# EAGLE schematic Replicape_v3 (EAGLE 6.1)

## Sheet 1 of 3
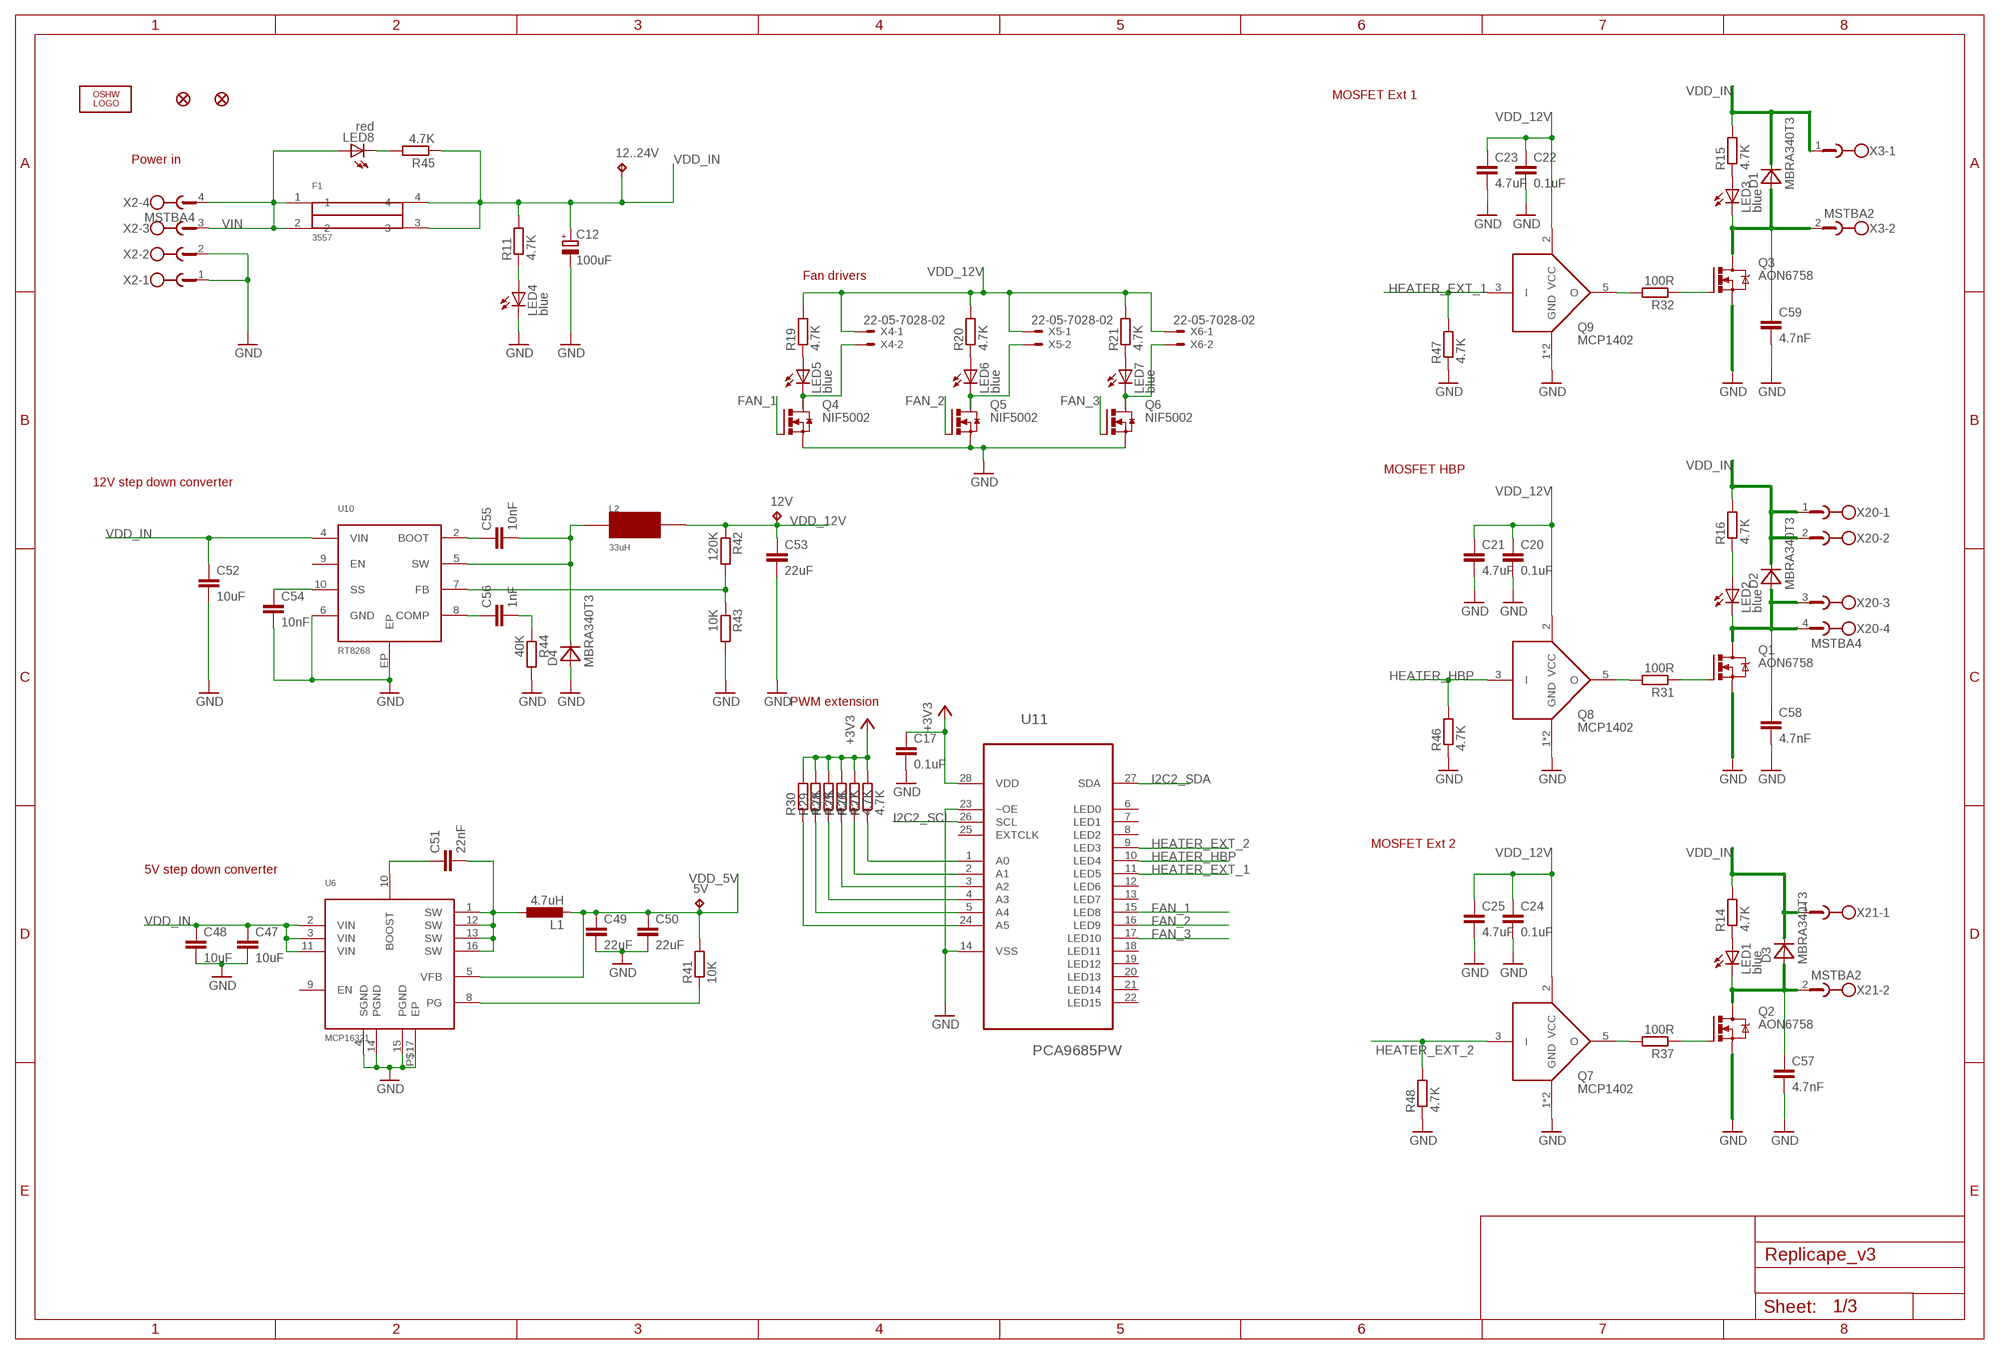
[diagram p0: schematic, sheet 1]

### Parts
5V  TPB1,27  [B1,27]
12..24V  TPB1,27  [B1,27]
12V  TPB1,27  [B1,27]
C12  100uF  CPOL-EU140CLH-0810  [140CLH-0810]
C17  0.1uF  C-EUC0402  [C0402]
C20  0.1uF  C-EUC0402  [C0402]
C21  4.7uF  C-EUC0402  [C0402]
C22  0.1uF  C-EUC0402  [C0402]
C23  4.7uF  C-EUC0402  [C0402]
C24  0.1uF  C-EUC0402  [C0402]
C25  4.7uF  C-EUC0402  [C0402]
C47  10uF  C-EUC1206  [C1206]
C48  10uF  C-EUC1206  [C1206]
C49  22uF  C-EUC0805  [C0805]
C50  22uF  C-EUC0805  [C0805]
C51  22nF  C-EUC0402  [C0402]
C52  10uF  C-EUC1206  [C1206]
C53  22uF  C-EUC0805  [C0805]
C54  10nF  C-EUC0402  [C0402]
C55  10nF  C-EUC0402  [C0402]
C56  1nF  C-EUC0402  [C0402]
C57  4.7nF  C-EUC0402  [C0402]
C58  4.7nF  C-EUC0402  [C0402]
C59  4.7nF  C-EUC0402  [C0402]
D1  MBRA340T3  [SMA]
D2  MBRA340T3  [SMA]
D3  MBRA340T3  [SMA]
D4  MBRA340T3  [SMA]
F1  3557  [3557]
JP1  FIDUCIAL1X2.5  [FIDUCIAL-1X2.5]
JP2  FIDUCIAL1X2.5  [FIDUCIAL-1X2.5]
L1  4.7uH  L-EUVLC  [VLC5020]
L2  33uH  RT8040T330  [NR8040T330]
LED1  blue  LEDCHIP-LED0603  [CHIP-LED0603]
LED2  blue  LEDCHIP-LED0603  [CHIP-LED0603]
LED3  blue  LEDCHIP-LED0603  [CHIP-LED0603]
LED4  blue  LEDCHIP-LED0603  [CHIP-LED0603]
LED5  blue  LEDCHIP-LED0603  [CHIP-LED0603]
LED6  blue  LEDCHIP-LED0603  [CHIP-LED0603]
LED7  blue  LEDCHIP-LED0603  [CHIP-LED0603]
LED8  red  LEDCHIP-LED0603  [CHIP-LED0603]
LOGO1  OSHW_LOGO_FILLX0200-NT  [OSHW_FILLX200_NOTEXT]
Q1  AON6758  [8-DFN-EP-(5X6)]
Q2  AON6758  [8-DFN-EP-(5X6)]
Q3  AON6758  [8-DFN-EP-(5X6)]
Q4  NIF5002  N-HEXFET-2D_SOT232-  [SOT223]
Q5  NIF5002  N-HEXFET-2D_SOT232-  [SOT223]
Q6  NIF5002  N-HEXFET-2D_SOT232-  [SOT223]
Q7  MCP1402  [SOT23-5L]
Q8  MCP1402  [SOT23-5L]
Q9  MCP1402  [SOT23-5L]
R11  4.7K  R-EU_R0402  [R0402]
R14  4.7K  R-EU_R0402  [R0402]
R15  4.7K  R-EU_R0402  [R0402]
R16  4.7K  R-EU_R0402  [R0402]
R19  4.7K  R-EU_R0402  [R0402]
R20  4.7K  R-EU_R0402  [R0402]
R21  4.7K  R-EU_R0402  [R0402]
R25  4.7K  R-EU_R0402  [R0402]
R26  4.7K  R-EU_R0402  [R0402]
R27  4.7K  R-EU_R0402  [R0402]
R28  4.7K  R-EU_R0402  [R0402]
R29  4.7K  R-EU_R0402  [R0402]
R30  4.7K  R-EU_R0402  [R0402]
R31  100R  R-EU_R0402  [R0402]
R32  100R  R-EU_R0402  [R0402]
R37  100R  R-EU_R0402  [R0402]
R41  10K  R-EU_R0402  [R0402]
R42  120K  R-EU_R0402  [R0402]
R43  10K  R-EU_R0402  [R0402]
R44  40K  R-EU_R0402  [R0402]
R45  4.7K  R-EU_R0402  [R0402]
R46  4.7K  R-EU_R0402  [R0402]
R47  4.7K  R-EU_R0402  [R0402]
R48  4.7K  R-EU_R0402  [R0402]
U6  MCP16321  [QFN-16]
U10  RT8268  [MSOP10]
U11  PCA9685PW  [SOP65P640X110-28N]
X2  MSTBA4  [MSTBA4]
X3  MSTBA2  [MSTBA2]
X4  22-05-7028-02  [7395-02]
X5  22-05-7028-02  [7395-02]
X6  22-05-7028-02  [7395-02]
X20  MSTBA4  [MSTBA4]
X21  MSTBA2  [MSTBA2]

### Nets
+3V3: C17.1 R25.2 R26.2 R27.2 R28.2 R29.2 R30.2 U11.28(VDD) ; also sheet 2,3
FAN_1: Q4.1(G) U11.15(LED8)
FAN_2: Q5.1(G) U11.16(LED9)
FAN_3: Q6.1(G) U11.17(LED10)
GND: C12.- C17.2 C20.2 C21.2 C22.2 C23.2 C24.2 C25.2 C47.2 C48.2 C49.2 C50.2 C52.2 C53.2 C54.2 C57.2 C58.2 C59.2 D4.A LED4.C Q1.1(S) Q1.2(S) Q1.3(S) Q2.1(S) Q2.2(S) Q2.3(S) Q3.1(S) Q3.2(S) Q3.3(S) Q4.3(S) Q5.3(S) Q6.3(S) Q7.1(GND) Q7.4(GND) Q8.1(GND) Q8.4(GND) Q9.1(GND) Q9.4(GND) R43.2 R44.2 R46.1 R47.1 R48.1 U6.4(SGND) U6.14(PGND) U6.15(PGND) U6.P$17(EP) U10.6(GND) U10.EP U11.14(VSS) U11.23(~OE) X2.1 X2.2 ; also sheet 2,3
HEATER_EXT_1: Q9.3(I) R47.2 U11.11(LED5)
HEATER_EXT_2: Q7.3(I) R48.2 U11.9(LED3)
HEATER_HBP: Q8.3(I) R46.2 U11.10(LED4)
I2C2_SCL: U11.26(SCL) ; also sheet 2
I2C2_SDA: U11.27(SDA) ; also sheet 2
N$8: LED8.C R45.2
N$9: LED5.A R19.1
N$21: Q9.5(O) R32.2
N$23: Q2.4(G) R37.1
N$41: Q7.5(O) R37.2
N$58: R27.1 U11.1(A0)
N$59: R26.1 U11.2(A1)
N$60: Q1.4(G) R31.1
N$61: Q8.5(O) R31.2
N$64: C57.1 D3.A LED1.C Q2.5(D) Q2.6(D) Q2.7(D) Q2.8(D) Q2.TH(D) X21.2
N$76: R25.1 U11.3(A2)
N$94: R28.1 U11.4(A3)
N$95: R29.1 U11.5(A4)
N$96: LED4.A R11.1
N$112: R30.1 U11.24(A5)
N$114: LED7.C Q6.2(D) Q6.4(D) X6.2
N$115: LED6.C Q5.2(D) Q5.4(D) X5.2
N$116: LED5.C Q4.2(D) Q4.4(D) X4.2
N$117: LED6.A R20.1
N$118: LED7.A R21.1
N$127: LED3.A R15.1
N$128: C51.1 U6.10(BOOST)
N$129: LED1.A R14.1
N$130: LED2.A R16.1
N$133: Q3.4(G) R32.1
N$233: R42.2 R43.1 U10.7(FB)
N$234: C59.1 D1.A LED3.C Q3.5(D) Q3.6(D) Q3.7(D) Q3.8(D) Q3.TH(D) X3.2
N$238: C55.2 D4.C L2.P$2 U10.5(SW)
N$239: R41.1 U6.8(PG)
N$242: C58.1 D2.A LED2.C Q1.5(D) Q1.6(D) Q1.7(D) Q1.8(D) Q1.TH(D) X20.3 X20.4
N$243: C54.1 U10.10(SS)
N$244: C56.1 U10.8(COMP)
N$245: C55.1 U10.2(BOOT)
N$246: C56.2 R44.1
SW: C51.2 L1.1 U6.1(SW) U6.12(SW) U6.13(SW) U6.16(SW)
VDD_5V: 5V.TP C49.1 C50.1 L1.2 R41.2 U6.5(VFB) ; also sheet 2
VDD_12V: 12V.TP C20.1 C21.1 C22.1 C23.1 C24.1 C25.1 C53.1 L2.P$1 Q7.2(VCC) Q8.2(VCC) Q9.2(VCC) R19.2 R20.2 R21.2 R42.1 X4.1 X5.1 X6.1
VDD_IN: 12..24V.TP C12.+ C47.1 C48.1 C52.1 D1.C D2.C D3.C F1.3 F1.4 R11.2 R14.2 R15.2 R16.2 R45.1 U6.2(VIN) U6.3(VIN) U6.11(VIN) U10.4(VIN) X3.1 X20.1 X20.2 X21.1 ; also sheet 3
VIN: F1.1 F1.2 LED8.A X2.3 X2.4
Unconnected: U6.9(EN) U10.9(EN) U11.6(LED0) U11.7(LED1) U11.8(LED2) U11.12(LED6) U11.13(LED7) U11.18(LED11) U11.19(LED12) U11.20(LED13) U11.21(LED14) U11.22(LED15) U11.25(EXTCLK)

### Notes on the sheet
- MOSFET Ext 1
- Power in
- Fan drivers
- MOSFET HBP
- 12V step down converter
- PWM extension
- MOSFET Ext 2
- 5V step down converter

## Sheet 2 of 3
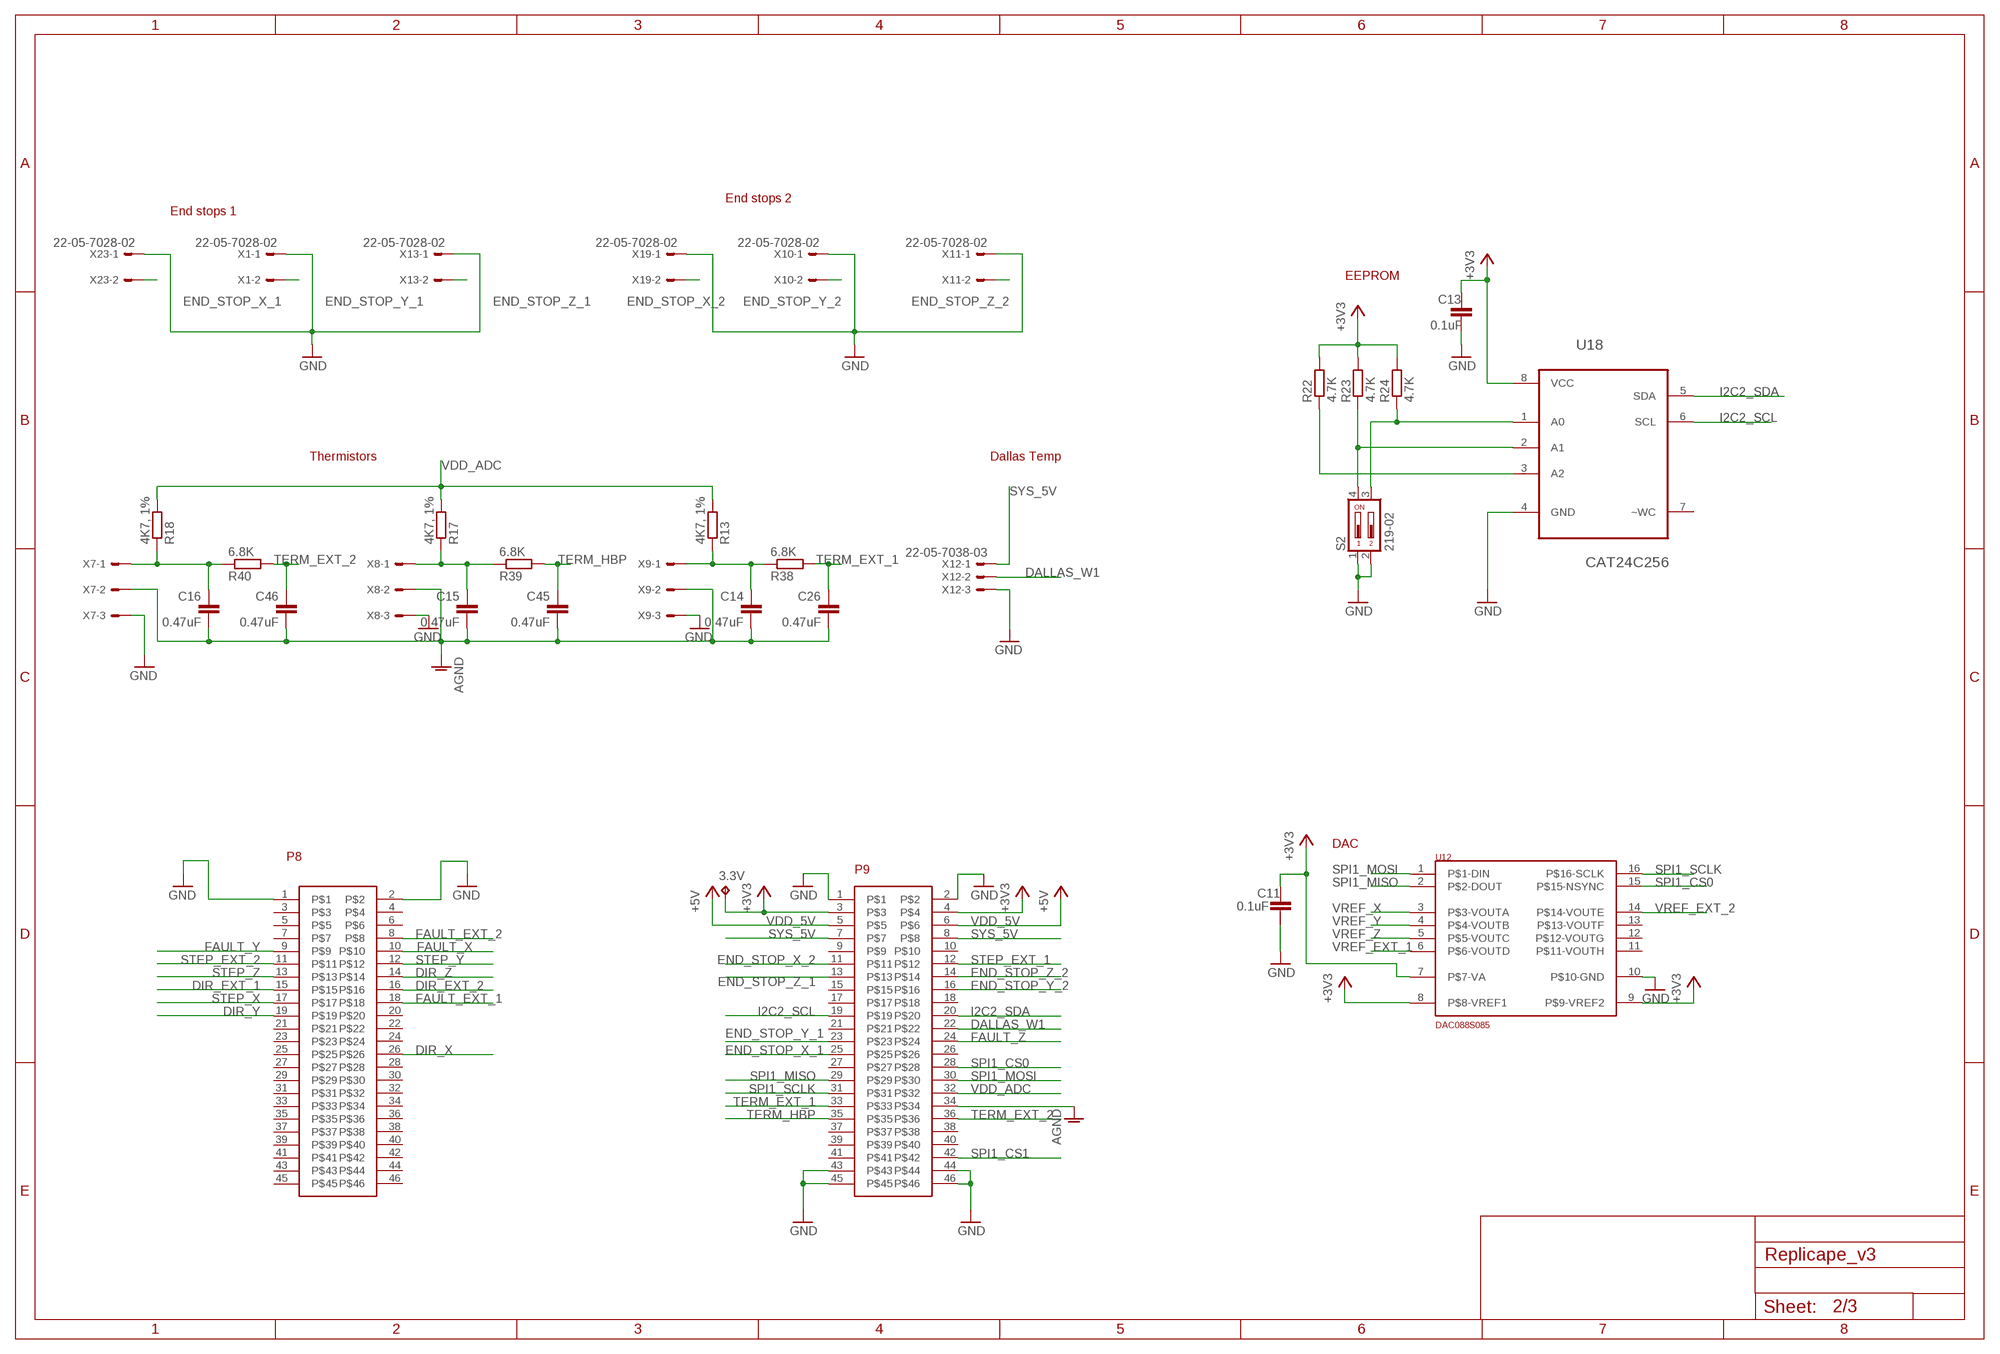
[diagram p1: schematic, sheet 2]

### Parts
3.3V  TPB1,27  [B1,27]
C11  0.1uF  C-EUC0402  [C0402]
C13  0.1uF  C-EUC0402  [C0402]
C14  0.47uF  C-EUC0402  [C0402]
C15  0.47uF  C-EUC0402  [C0402]
C16  0.47uF  C-EUC0402  [C0402]
C26  0.47uF  C-EUC0402  [C0402]
C45  0.47uF  C-EUC0402  [C0402]
C46  0.47uF  C-EUC0402  [C0402]
P9-EXPANSION_A  BEAGLE_EXT9  [2X23]
P9-EXPANSION_A1  BEAGLE_EXT9  [2X23]
R13  4K7, 1%  R-EU_R0402  [R0402]
R17  4K7, 1%  R-EU_R0402  [R0402]
R18  4K7, 1%  R-EU_R0402  [R0402]
R22  4.7K  R-EU_R0402  [R0402]
R23  4.7K  R-EU_R0402  [R0402]
R24  4.7K  R-EU_R0402  [R0402]
R38  6.8K  R-EU_R0402  [R0402]
R39  6.8K  R-EU_R0402  [R0402]
R40  6.8K  R-EU_R0402  [R0402]
S2  219-02  [CTS-219-02]
U12  DAC088S085  [TSSOP-16]
U18  CAT24C256  [SOIC127P600X175-8N]
X1  22-05-7028-02  [7395-02]
X7  22-05-7038-03  [7395-03]
X8  22-05-7038-03  [7395-03]
X9  22-05-7038-03  [7395-03]
X10  22-05-7028-02  [7395-02]
X11  22-05-7028-02  [7395-02]
X12  22-05-7038-03  [7395-03]
X13  22-05-7028-02  [7395-02]
X19  22-05-7028-02  [7395-02]
X23  22-05-7028-02  [7395-02]

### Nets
+3V3: 3.3V.TP C11.1 C13.1 P9-EXPANSION_A.3 P9-EXPANSION_A.4 R22.2 R23.2 R24.2 U12.7(P$7-VA) U12.8(P$8-VREF1) U12.9(P$9-VREF2) U18.8(VCC) ; also sheet 1,3
AGND: C14.2 C15.2 C16.2 C26.2 C45.2 C46.2 P9-EXPANSION_A.34 X7.2 X8.2 X9.2
DALLAS_W1: P9-EXPANSION_A.22 X12.2
DIR_EXT_1: P9-EXPANSION_A1.15 ; also sheet 3
DIR_EXT_2: P9-EXPANSION_A1.16 ; also sheet 3
DIR_X: P9-EXPANSION_A1.26 ; also sheet 3
DIR_Y: P9-EXPANSION_A1.19 ; also sheet 3
DIR_Z: P9-EXPANSION_A1.14 ; also sheet 3
END_STOP_X_1: P9-EXPANSION_A.25 X23.2
END_STOP_X_2: P9-EXPANSION_A.11 X19.2
END_STOP_Y_1: P9-EXPANSION_A.23 X1.2
END_STOP_Y_2: P9-EXPANSION_A.16 X10.2
END_STOP_Z_1: P9-EXPANSION_A.13 X13.2
END_STOP_Z_2: P9-EXPANSION_A.14 X11.2
FAULT_EXT_1: P9-EXPANSION_A1.18 ; also sheet 3
FAULT_EXT_2: P9-EXPANSION_A1.8 ; also sheet 3
FAULT_X: P9-EXPANSION_A1.10 ; also sheet 3
FAULT_Y: P9-EXPANSION_A1.9 ; also sheet 3
FAULT_Z: P9-EXPANSION_A.24 ; also sheet 3
GND: C11.2 C13.2 P9-EXPANSION_A1.1 P9-EXPANSION_A1.2 P9-EXPANSION_A.1 P9-EXPANSION_A.2 P9-EXPANSION_A.43 P9-EXPANSION_A.44 P9-EXPANSION_A.45 P9-EXPANSION_A.46 S2.1 S2.2 U12.10(P$10-GND) U18.4(GND) X1.1 X7.3 X8.3 X9.3 X10.1 X11.1 X12.3 X13.1 X19.1 X23.1 ; also sheet 1,3
I2C2_SCL: P9-EXPANSION_A.19 U18.6(SCL) ; also sheet 1
I2C2_SDA: P9-EXPANSION_A.20 U18.5(SDA) ; also sheet 1
N$147: R24.1 S2.3 U18.1(A0)
N$148: R23.1 S2.4 U18.2(A1)
N$149: R22.1 U18.3(A2)
N$237: C14.1 R13.1 R38.1 X9.1
N$240: C16.1 R18.1 R40.1 X7.1
N$241: C15.1 R17.1 R39.1 X8.1
SPI1_CS0: P9-EXPANSION_A.28 U12.15(P$15-NSYNC)
SPI1_CS1: P9-EXPANSION_A.42 ; also sheet 3
SPI1_MISO: P9-EXPANSION_A.29 U12.2(P$2-DOUT)
SPI1_MOSI: P9-EXPANSION_A.30 U12.1(P$1-DIN) ; also sheet 3
SPI1_SCLK: P9-EXPANSION_A.31 U12.16(P$16-SCLK) ; also sheet 3
STEP_EXT_1: P9-EXPANSION_A.12 ; also sheet 3
STEP_EXT_2: P9-EXPANSION_A1.11 ; also sheet 3
STEP_X: P9-EXPANSION_A1.17 ; also sheet 3
STEP_Y: P9-EXPANSION_A1.12 ; also sheet 3
STEP_Z: P9-EXPANSION_A1.13 ; also sheet 3
SYS_5V: P9-EXPANSION_A.7 P9-EXPANSION_A.8 X12.1
TERM_EXT_1: C26.1 P9-EXPANSION_A.33 R38.2
TERM_EXT_2: C46.1 P9-EXPANSION_A.36 R40.2
TERM_HBP: C45.1 P9-EXPANSION_A.35 R39.2
VDD_5V: P9-EXPANSION_A.5 P9-EXPANSION_A.6 ; supply symbol labelled +5V ; also sheet 1
VDD_ADC: P9-EXPANSION_A.32 R13.2 R17.2 R18.2
VREF_EXT_1: U12.6(P$6-VOUTD) ; also sheet 3
VREF_EXT_2: U12.14(P$14-VOUTE) ; also sheet 3
VREF_X: U12.3(P$3-VOUTA) ; also sheet 3
VREF_Y: U12.4(P$4-VOUTB) ; also sheet 3
VREF_Z: U12.5(P$5-VOUTC) ; also sheet 3
Unconnected: P9-EXPANSION_A1.3 P9-EXPANSION_A1.4 P9-EXPANSION_A1.5 P9-EXPANSION_A1.6 P9-EXPANSION_A1.7 P9-EXPANSION_A1.20 P9-EXPANSION_A1.21 P9-EXPANSION_A1.22 P9-EXPANSION_A1.23 P9-EXPANSION_A1.24 P9-EXPANSION_A1.25 P9-EXPANSION_A1.27 P9-EXPANSION_A1.28 P9-EXPANSION_A1.29 P9-EXPANSION_A1.30 P9-EXPANSION_A1.31 P9-EXPANSION_A1.32 P9-EXPANSION_A1.33 P9-EXPANSION_A1.34 P9-EXPANSION_A1.35 P9-EXPANSION_A1.36 P9-EXPANSION_A1.37 P9-EXPANSION_A1.38 P9-EXPANSION_A1.39 P9-EXPANSION_A1.40 P9-EXPANSION_A1.41 P9-EXPANSION_A1.42 P9-EXPANSION_A1.43 P9-EXPANSION_A1.44 P9-EXPANSION_A1.45 P9-EXPANSION_A1.46 P9-EXPANSION_A.9 P9-EXPANSION_A.10 P9-EXPANSION_A.15 P9-EXPANSION_A.17 P9-EXPANSION_A.18 P9-EXPANSION_A.21 P9-EXPANSION_A.26 P9-EXPANSION_A.27 P9-EXPANSION_A.37 P9-EXPANSION_A.38 P9-EXPANSION_A.39 P9-EXPANSION_A.40 P9-EXPANSION_A.41 U12.11(P$11-VOUTH) U12.12(P$12-VOUTG) U12.13(P$13-VOUTF) U18.7(~WC)

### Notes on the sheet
- End stops 2
- End stops 1
- EEPROM
- Thermistors | Dallas Temp
- DAC
- P8
- P9

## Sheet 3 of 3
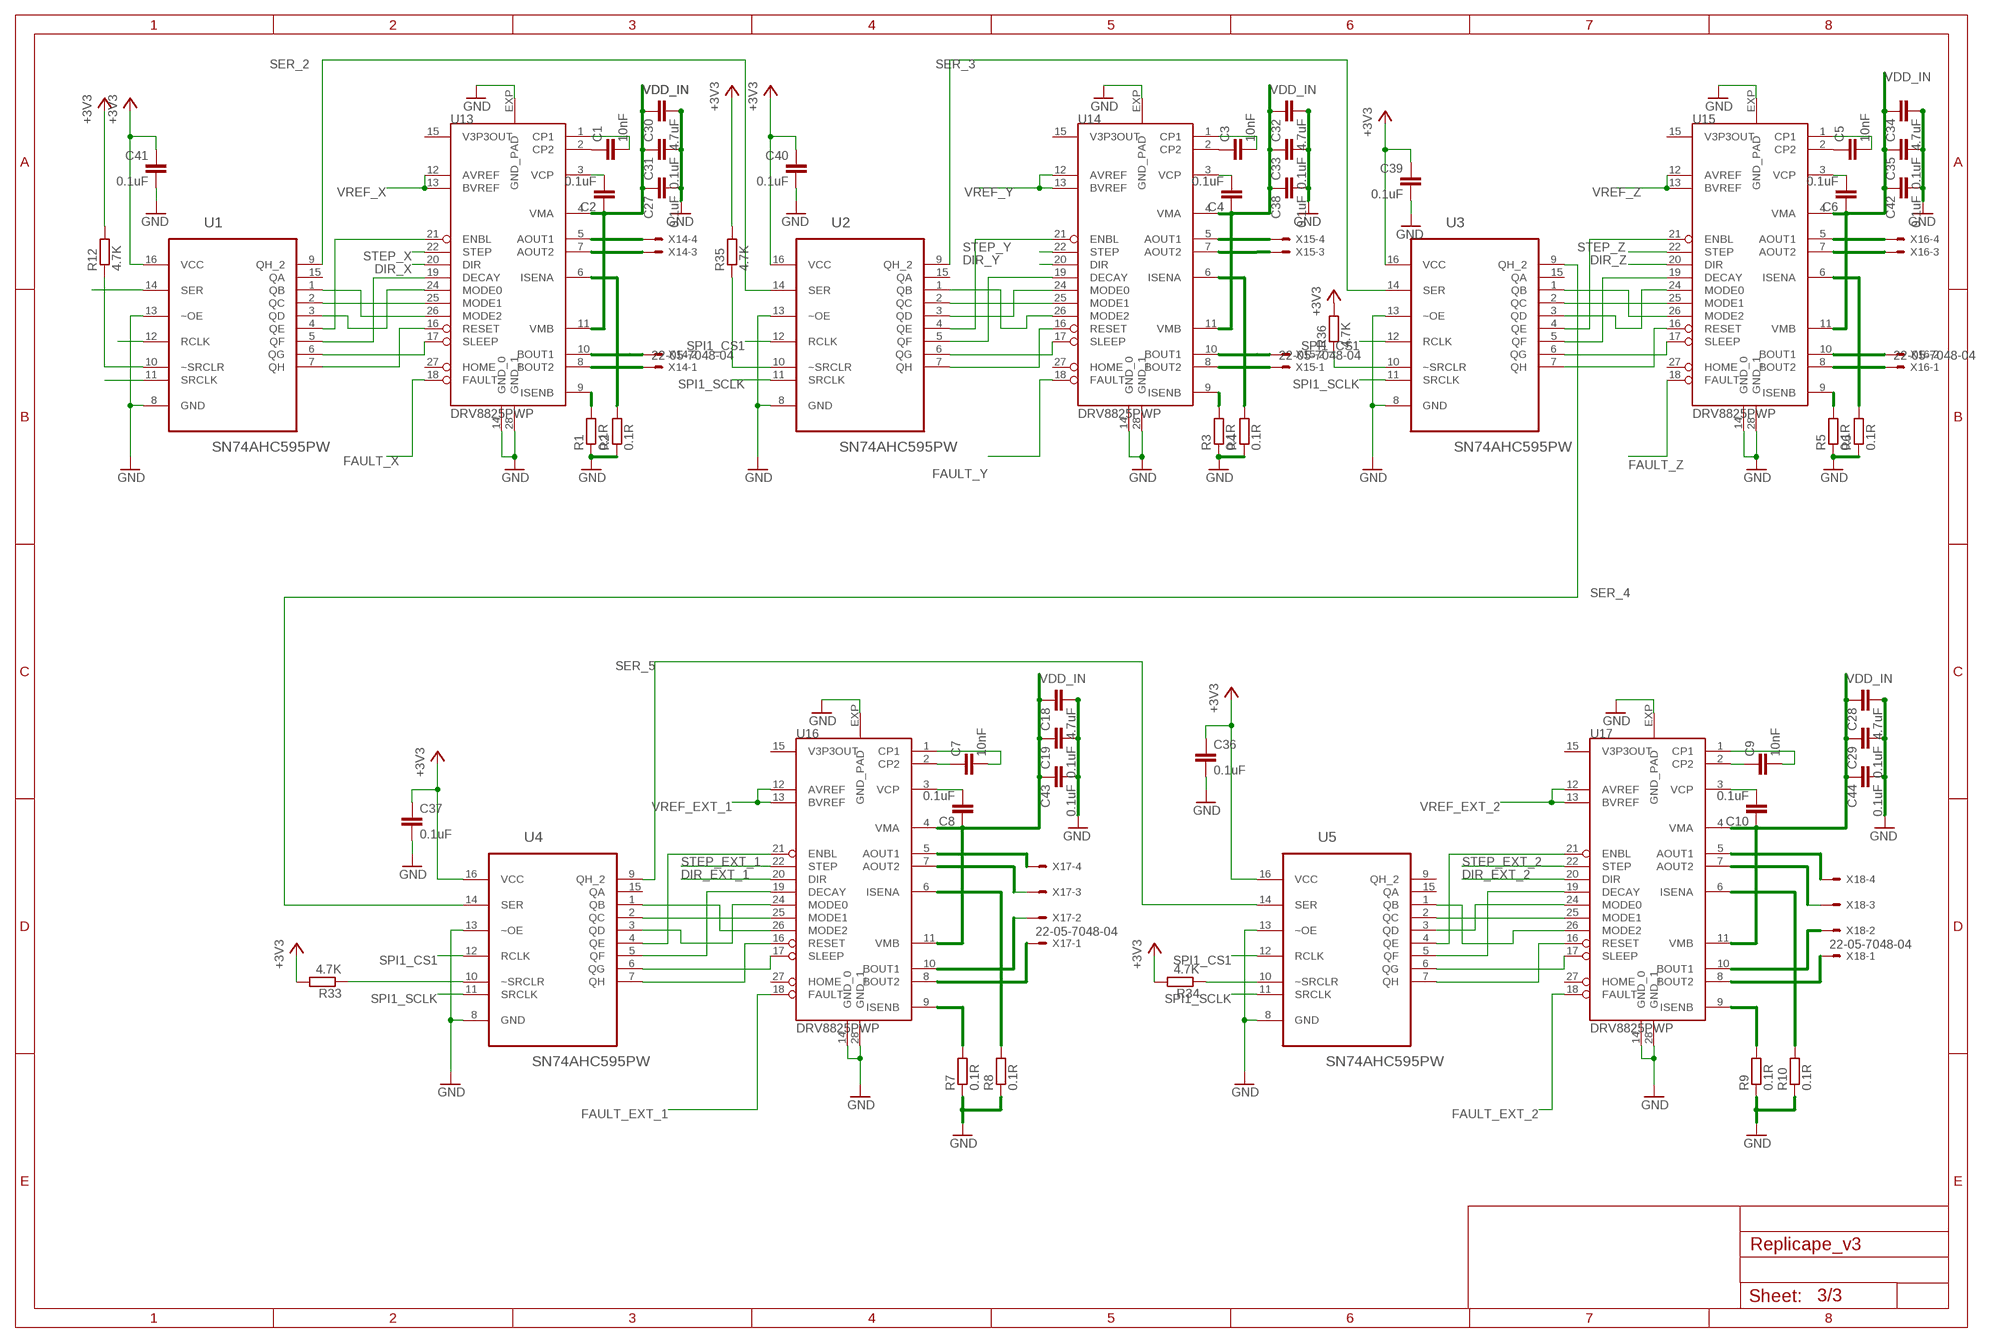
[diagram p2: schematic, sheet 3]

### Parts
C1  10nF  C-EUC0402  [C0402]
C2  0.1uF  C-EUC0402  [C0402]
C3  10nF  C-EUC0402  [C0402]
C4  0.1uF  C-EUC0402  [C0402]
C5  10nF  C-EUC0402  [C0402]
C6  0.1uF  C-EUC0402  [C0402]
C7  10nF  C-EUC0402  [C0402]
C8  0.1uF  C-EUC0402  [C0402]
C9  10nF  C-EUC0402  [C0402]
C10  0.1uF  C-EUC0402  [C0402]
C18  4.7uF  C-EUC0603  [C0603]
C19  0.1uF  C-EUC0402  [C0402]
C27  0.1uF  C-EUC0402  [C0402]
C28  4.7uF  C-EUC0603  [C0603]
C29  0.1uF  C-EUC0402  [C0402]
C30  4.7uF  C-EUC0603  [C0603]
C31  0.1uF  C-EUC0402  [C0402]
C32  4.7uF  C-EUC0603  [C0603]
C33  0.1uF  C-EUC0402  [C0402]
C34  4.7uF  C-EUC0603  [C0603]
C35  0.1uF  C-EUC0402  [C0402]
C36  0.1uF  C-EUC0402  [C0402]
C37  0.1uF  C-EUC0402  [C0402]
C38  0.1uF  C-EUC0402  [C0402]
C39  0.1uF  C-EUC0402  [C0402]
C40  0.1uF  C-EUC0402  [C0402]
C41  0.1uF  C-EUC0402  [C0402]
C42  0.1uF  C-EUC0402  [C0402]
C43  0.1uF  C-EUC0402  [C0402]
C44  0.1uF  C-EUC0402  [C0402]
R1  0.1R  R-EU_R0805  [R0805]
R2  0.1R  R-EU_R0805  [R0805]
R3  0.1R  R-EU_R0805  [R0805]
R4  0.1R  R-EU_R0805  [R0805]
R5  0.1R  R-EU_R0805  [R0805]
R6  0.1R  R-EU_R0805  [R0805]
R7  0.1R  R-EU_R0805  [R0805]
R8  0.1R  R-EU_R0805  [R0805]
R9  0.1R  R-EU_R0805  [R0805]
R10  0.1R  R-EU_R0805  [R0805]
R12  4.7K  R-EU_R0402  [R0402]
R33  4.7K  R-EU_R0402  [R0402]
R34  4.7K  R-EU_R0402  [R0402]
R35  4.7K  R-EU_R0402  [R0402]
R36  4.7K  R-EU_R0402  [R0402]
U1  SN74AHC595PW  [SOP65P640X120-16N]
U2  SN74AHC595PW  [SOP65P640X120-16N]
U3  SN74AHC595PW  [SOP65P640X120-16N]
U4  SN74AHC595PW  [SOP65P640X120-16N]
U5  SN74AHC595PW  [SOP65P640X120-16N]
U13  DRV8825PWP  [TSSOP-28]
U14  DRV8825PWP  [TSSOP-28]
U15  DRV8825PWP  [TSSOP-28]
U16  DRV8825PWP  [TSSOP-28]
U17  DRV8825PWP  [TSSOP-28]
X14  22-05-7048-04  [7395-04]
X15  22-05-7048-04  [7395-04]
X16  22-05-7048-04  [7395-04]
X17  22-05-7048-04  [7395-04]
X18  22-05-7048-04  [7395-04]

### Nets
+3V3: C36.1 C37.1 C39.1 C40.1 C41.1 R12.2 R33.2 R34.2 R35.2 R36.2 U1.16(VCC) U2.16(VCC) U3.16(VCC) U4.16(VCC) U5.16(VCC) ; also sheet 1,2
DIR_EXT_1: U16.20(DIR) ; also sheet 2
DIR_EXT_2: U17.20(DIR) ; also sheet 2
DIR_X: U13.20(DIR) ; also sheet 2
DIR_Y: U14.20(DIR) ; also sheet 2
DIR_Z: U15.20(DIR) ; also sheet 2
EXT1_NENABLE: U4.4(QE) U16.21(ENBL)
EXT1_NSLEEP: U4.6(QG) U16.17(SLEEP)
FAULT_EXT_1: U16.18(FAULT) ; also sheet 2
FAULT_EXT_2: U17.18(FAULT) ; also sheet 2
FAULT_X: U13.18(FAULT) ; also sheet 2
FAULT_Y: U14.18(FAULT) ; also sheet 2
FAULT_Z: U15.18(FAULT) ; also sheet 2
GND: C18.2 C19.2 C27.2 C28.2 C29.2 C30.2 C31.2 C32.2 C33.2 C34.2 C35.2 C36.2 C37.2 C38.2 C39.2 C40.2 C41.2 C42.2 C43.2 C44.2 R1.1 R2.1 R3.1 R4.1 R5.1 R6.1 R7.1 R8.1 R9.1 R10.1 U1.8(GND) U1.13(~OE) U2.8(GND) U2.13(~OE) U3.8(GND) U3.13(~OE) U4.8(GND) U4.13(~OE) U5.8(GND) U5.13(~OE) U13.14(GND_0) U13.28(GND_1) U13.EXP(GND_PAD) U14.14(GND_0) U14.28(GND_1) U14.EXP(GND_PAD) U15.14(GND_0) U15.28(GND_1) U15.EXP(GND_PAD) U16.14(GND_0) U16.28(GND_1) U16.EXP(GND_PAD) U17.14(GND_0) U17.28(GND_1) U17.EXP(GND_PAD) ; also sheet 1,2
N$1: U5.1(QB) U17.26(MODE2)
N$2: U5.3(QD) U17.24(MODE0)
N$3: U5.7(QH) U17.16(RESET)
N$4: U4.7(QH) U16.16(RESET)
N$5: U4.3(QD) U16.24(MODE0)
N$6: U4.1(QB) U16.26(MODE2)
N$7: U3.7(QH) U15.16(RESET)
N$11: U3.3(QD) U15.24(MODE0)
N$12: U3.1(QB) U15.26(MODE2)
N$13: U2.7(QH) U14.16(RESET)
N$14: U2.1(QB) U14.26(MODE2)
N$15: U2.3(QD) U14.24(MODE0)
N$16: C1.1 U13.2(CP2)
N$17: C1.2 U13.1(CP1)
N$18: R1.2 U13.9(ISENB)
N$19: R2.2 U13.6(ISENA)
N$20: U1.7(QH) U13.16(RESET)
N$22: C2.2 U13.3(VCP)
N$24: U1.1(QB) U13.26(MODE2)
N$25: U1.3(QD) U13.24(MODE0)
N$26: U2.5(QF) U14.19(DECAY)
N$27: U3.5(QF) U15.19(DECAY)
N$28: U5.5(QF) U17.19(DECAY)
N$29: U4.5(QF) U16.19(DECAY)
N$34: C3.1 U14.2(CP2)
N$35: C3.2 U14.1(CP1)
N$36: R3.2 U14.9(ISENB)
N$37: R4.2 U14.6(ISENA)
N$38: C4.2 U14.3(VCP)
N$52: C5.1 U15.2(CP2)
N$53: C5.2 U15.1(CP1)
N$54: R5.2 U15.9(ISENB)
N$55: R6.2 U15.6(ISENA)
N$56: C6.2 U15.3(VCP)
N$62: U4.2(QC) U16.25(MODE1)
N$70: C7.1 U16.2(CP2)
N$71: C7.2 U16.1(CP1)
N$72: R7.2 U16.9(ISENB)
N$73: R8.2 U16.6(ISENA)
N$74: C8.2 U16.3(VCP)
N$80: U5.2(QC) U17.25(MODE1)
N$83: U5.6(QG) U17.17(SLEEP)
N$88: C9.1 U17.2(CP2)
N$89: C9.2 U17.1(CP1)
N$90: R9.2 U17.9(ISENB)
N$91: R10.2 U17.6(ISENA)
N$92: C10.2 U17.3(VCP)
N$93: U5.4(QE) U17.21(ENBL)
N$97: R12.1 U1.10(~SRCLR)
N$98: R33.1 U4.10(~SRCLR)
N$99: R34.1 U5.10(~SRCLR)
N$100: R35.1 U2.10(~SRCLR)
N$101: R36.1 U3.10(~SRCLR)
SER_2: U1.9(QH_2) U2.14(SER)
SER_3: U2.9(QH_2) U3.14(SER)
SER_4: U3.9(QH_2) U4.14(SER)
SER_5: U4.9(QH_2) U5.14(SER)
SPI1_CS1: U1.12(RCLK) U2.12(RCLK) U3.12(RCLK) U4.12(RCLK) U5.12(RCLK) ; also sheet 2
SPI1_MOSI: U1.14(SER) ; also sheet 2
SPI1_SCLK: U1.11(SRCLK) U2.11(SRCLK) U3.11(SRCLK) U4.11(SRCLK) U5.11(SRCLK) ; also sheet 2
STEP1_EXT1: U16.5(AOUT1) X17.4
STEP1_EXT2: U17.5(AOUT1) X18.4
STEP1_X: U13.5(AOUT1) X14.4
STEP1_Y: U14.5(AOUT1) X15.4
STEP1_Z: U15.5(AOUT1) X16.4
STEP2_EXT1: U16.7(AOUT2) X17.3
STEP2_EXT2: U17.7(AOUT2) X18.3
STEP2_X: U13.7(AOUT2) X14.3
STEP2_Y: U14.7(AOUT2) X15.3
STEP2_Z: U15.7(AOUT2) X16.3
STEP3_EXT1: U16.10(BOUT1) X17.2
STEP3_EXT2: U17.10(BOUT1) X18.2
STEP3_X: U13.10(BOUT1) X14.2
STEP3_Y: U14.10(BOUT1) X15.2
STEP3_Z: U15.10(BOUT1) X16.2
STEP4_EXT1: U16.8(BOUT2) X17.1
STEP4_EXT2: U17.8(BOUT2) X18.1
STEP4_X: U13.8(BOUT2) X14.1
STEP4_Y: U14.8(BOUT2) X15.1
STEP4_Z: U15.8(BOUT2) X16.1
STEP_EXT_1: U16.22(STEP) ; also sheet 2
STEP_EXT_2: U17.22(STEP) ; also sheet 2
STEP_X: U13.22(STEP) ; also sheet 2
STEP_Y: U14.22(STEP) ; also sheet 2
STEP_Z: U15.22(STEP) ; also sheet 2
VDD_IN: C2.1 C4.1 C6.1 C8.1 C10.1 C18.1 C19.1 C27.1 C28.1 C29.1 C30.1 C31.1 C32.1 C33.1 C34.1 C35.1 C38.1 C42.1 C43.1 C44.1 U13.4(VMA) U13.11(VMB) U14.4(VMA) U14.11(VMB) U15.4(VMA) U15.11(VMB) U16.4(VMA) U16.11(VMB) U17.4(VMA) U17.11(VMB) ; also sheet 1
VREF_EXT_1: U16.12(AVREF) U16.13(BVREF) ; also sheet 2
VREF_EXT_2: U17.12(AVREF) U17.13(BVREF) ; also sheet 2
VREF_X: U13.12(AVREF) U13.13(BVREF) ; also sheet 2
VREF_Y: U14.12(AVREF) U14.13(BVREF) ; also sheet 2
VREF_Z: U15.12(AVREF) U15.13(BVREF) ; also sheet 2
X_DECAY: U1.5(QF) U13.19(DECAY)
X_ENABLE: U1.4(QE) U13.21(ENBL)
X_MODE1: U1.2(QC) U13.25(MODE1)
X_SLEEP: U1.6(QG) U13.17(SLEEP)
Y_ENABLE: U2.4(QE) U14.21(ENBL)
Y_MODE1: U2.2(QC) U14.25(MODE1)
Y_SLEEP: U2.6(QG) U14.17(SLEEP)
Z_ENABLE: U3.4(QE) U15.21(ENBL)
Z_MODE1: U3.2(QC) U15.25(MODE1)
Z_SLEEP: U3.6(QG) U15.17(SLEEP)
Unconnected: U1.15(QA) U2.15(QA) U3.15(QA) U4.15(QA) U5.9(QH_2) U5.15(QA) U13.15(V3P3OUT) U13.27(HOME) U14.15(V3P3OUT) U14.27(HOME) U15.15(V3P3OUT) U15.27(HOME) U16.15(V3P3OUT) U16.27(HOME) U17.15(V3P3OUT) U17.27(HOME)

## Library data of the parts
3.3V 5V 12..24V 12V = testpad:TP: Test pad
C1-C11 C13-C59 = rcl:C-EU: CAPACITOR, European symbol
C12 = rcl:CPOL-EU: POLARIZED CAPACITOR, European symbol
D1-D4 = diode:MBRA340T3: Surface Mount Schottky Power Rectifier
F1 = SparkFun:3557
JP1 JP2 = SparkFun:FIDUCIAL: Fiducial Alignment Points
L1 = resistor:L-EU: INDUCTOR, European symbol
L2 = SparkFun:RT8040T330
LED1-LED8 = led:LED: LED
LOGO1 = ohw-logo:OSHW_LOGO_FILL
P9-EXPANSION_A P9-EXPANSION_A1 = custom:BEAGLE_EXT9
Q1-Q3 = transistor-power:AON6758
Q4-Q6 = transistor-power:N-HEXFET-2D_?-*: HEXFET® Power MOSFET 2 Drain connects http://www.irf.com/product-info/datasheets/data/irll014n.pdf
Q7-Q9 = microchip-6:MCP1402: MOSFET driver
R1-R48 = rcl:R-EU_: RESISTOR, European symbol
S2 = switch-dil:219-02*: Surface Mount DIP Switch Series 219 SMT CTS Electronic Components Sourc: www.ctscorp.com; OC_FARNELL: unknown; OC_NEWARK: unknown
U1-U5 = sn74hc595:SN74AHC595PW: 8 bit shift registers with 3-state output registers; MPN: SN74AHC595PW; OC_FARNELL: 1741463; OC_NEWARK: 50R5930; PACKAGE: TSSOP-16; SUPPLIER: Texas Instruments
U6 = SparkFun:MCP16321
U10 = SparkFun:RT8268
U11 = custom:PCA9685PW: 16-channel, 12-bit PWM Fm+ I2C-bus LED controller; MPN: PCA9685PW; OC_FARNELL: 1854074; OC_NEWARK: 19T6398; PACKAGE: TSSOP-28; SUPPLIER: NXP
U12 = dac88s:DAC088S085
U13-U17 = drv88xx:DRV8825PWP
U18 = custom:CAT24C256
X1 X4-X6 X10 X11 X13 X19 X23 = con-molex:22-?-02: CONNECTOR; OC_FARNELL: 9731601; OC_NEWARK: unknown
X2 X20 = con-phoenix-508:MSTBA4: PHOENIX
X3 X21 = con-phoenix-508:MSTBA2: PHOENIX
X7-X9 X12 = con-molex:22-?-03: CONNECTOR wire to board 2.54 mm (.1 inch) pitch header; OC_FARNELL: unknown; OC_NEWARK: unknown
X14-X18 = con-molex:22-?-04: CONNECTOR wire to board 2.54 mm (.1 inch) pitch header; OC_FARNELL: unknown; OC_NEWARK: unknown

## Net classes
1 power: width 1.27 mm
